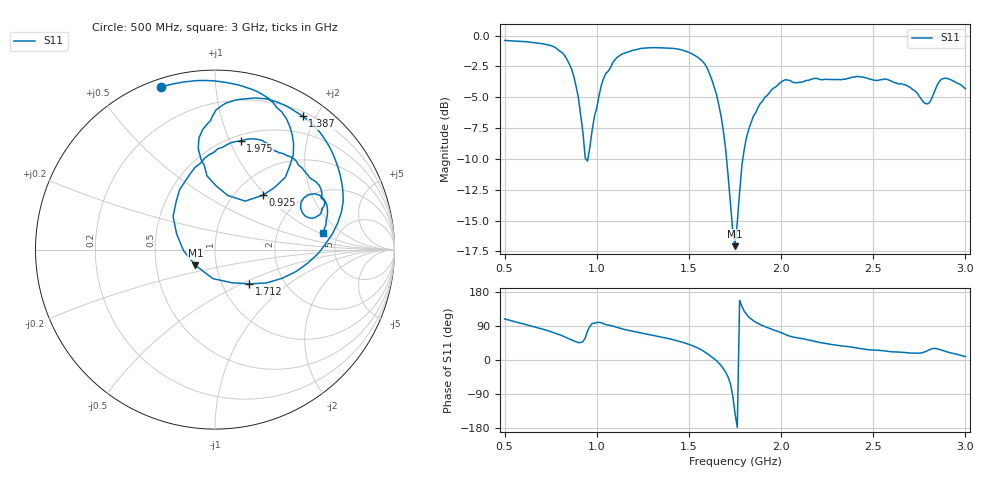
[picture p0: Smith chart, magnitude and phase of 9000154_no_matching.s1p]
#  HZ  S  DB  R  50.00
! Rohde & Schwarz Vector Network Analyzer
! Rohde-Schwarz,ZNB8-4Port,1311601044101844,3.45
! Created: UTC 10/4/2024, 7:17:57 AM
! freq[Hz]  db:S22  ang:S22
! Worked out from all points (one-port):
!   201 points, 500 MHz to 3 GHz, reference 50 ohm
!   lowest |S11| = -17.1 dB at 1.75 GHz (marker M1), VSWR 1.33, Z = 39.6 - j7.12 ohm
!   |S11| at or under -10 dB: 940.4 MHz to 952 MHz (11.57 MHz wide, 1.22 % of centre); 1.704 GHz to 1.793 GHz (88.35 MHz wide, 5.05 % of centre)
!   S11 on the Smith chart (normalised r, x): 500 MHz: 0.03, +0.72; 925 MHz: 1.33, +0.97; 1.387 GHz: 0.26, +1.83; 1.712 GHz: 1.34, -0.55; 1.975 GHz: 0.56, +1.10; 3 GHz: 3.75, +1.13
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5e8  -0.40 108.4
7e8  -0.66 82.4
8.125e8  -1.39 64.0
8.75e8  -3.29 50.5
9.25e8  -7.86 48.6
9.5e8  -10.18 76.5
9.75e8  -7.67 96.2
1.0125e9  -4.85 99.4
1.125e9  -1.62 83.8
1.25e9  -1.03 70.4
1.3875e9  -1.02 56.7
1.4375e9  -1.09 50.6
1.5375e9  -1.66 34.1
1.6e9  -2.68 16.5
1.65e9  -4.80 -2.2
1.7125e9  -11.35 -44.9
1.75e9  -17.08 -141.0
1.7875e9  -10.51 141.6
1.8125e9  -8.24 120.6
1.8875e9  -5.51 93.3
1.975e9  -4.12 76.7
2.0625e9  -3.79 60.6
2.375e9  -3.43 34.6
2.6875e9  -4.10 19.1
2.8e9  -5.51 26.0
2.85e9  -3.93 29.3
2.9e9  -3.47 21.5
3e9  -4.31 8.9
